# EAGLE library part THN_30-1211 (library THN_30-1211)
30 Watt DC/DC converter, industrial, 2:1 input, encpasulated, 1.0" x 1.0" metal package Source: Datasheet
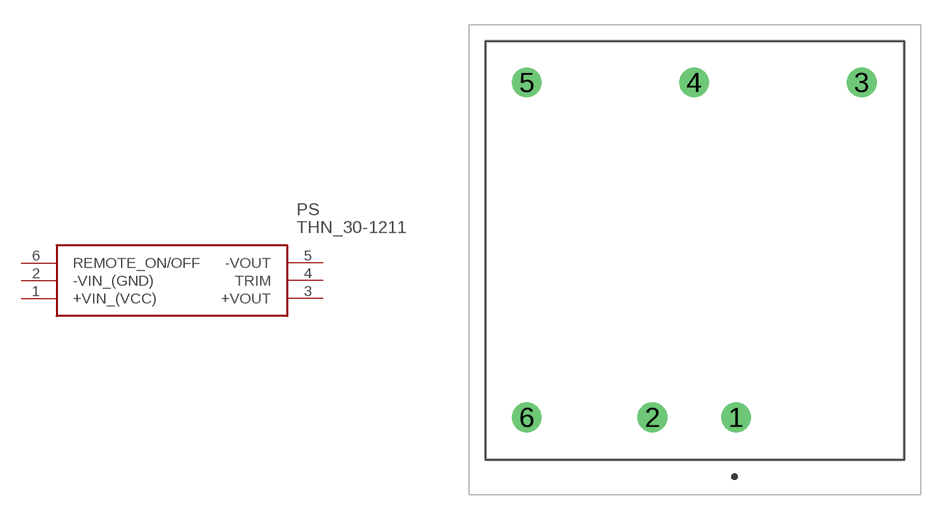
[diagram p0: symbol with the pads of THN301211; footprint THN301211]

Designator prefix PS

## THN_30-1211 (Description: 30 Watt DC/DC converter, industrial, 2:1 input, encpasulated, 1.0" x 1.0" metal package; Height: 10.4mm; Manufacturer_Name: Traco Power; Manufacturer_Part_Number: THN 30-1211; Mouser_Part_Number: 495-THN-30-1211; Mouser_Price-Stock: https://www.mouser.co.uk/ProductDetail/TRACO-Power/THN-30-1211?qs=ckJk83FOD0XjmIpWKdS%252Buw%3D%3D)  [THN301211]
1  +VIN_(VCC)
2  -VIN_(GND)
3  +VOUT
4  TRIM
5  -VOUT
6  REMOTE_ON/OFF

## Footprint THN301211 (pad centres in mm)
THN 30-1211-1
drill 1.2 pad 1.8: 1 0,0; 2 -5.08,0; 3 7.62,20.32; 4 -2.54,20.32; 5 -12.7,20.32; 6 -12.7,0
